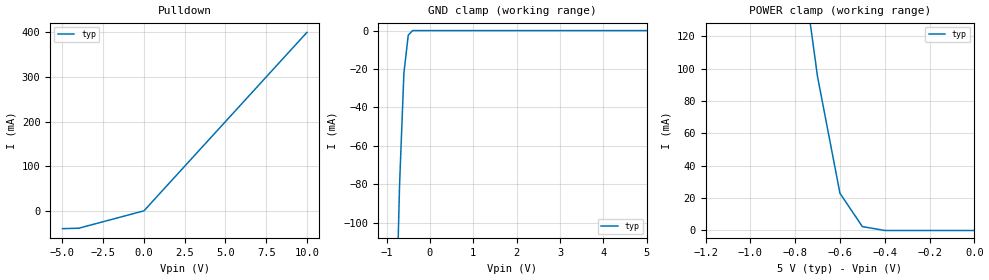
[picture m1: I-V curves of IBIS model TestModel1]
[IBIS Ver]   3.2
[File Name]   bug54b.ibs
[File Rev]   0.0
[Date]   22-February-2001
[Source]   File created from specification
[Notes]   Using the IBISCHK3 v3.2.5 & v3.2.6 parsers, the
   following file will show two misleading warnings
   related to the buffer delay fixture.
[Disclaimer]
   (C) Copyright 2001 Intel Corp.
   All rights reserved
   This model is for demonstration purposes only,
[Component]   GENERIC_IBIS
[Manufacturer]   Intel Corp.
[Package]
|   typ   min   max
R_pkg   6.0mO   5.0mO   7.0mO
L_pkg   5.0nH   2.0nH   8.0nH
C_pkg   1.0pF   0.5pF   1.5pF
[Pin]   signal_name   model_name   R_pin   L_pin   C_pin
   1   TestSignal1   TestModel1
| Models and submodels in the file (1): TestModel1 (I/O_open_sink)
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[Model]   TestModel1
Model_type   I/O_open_sink
| Model_type   I/O
Polarity   Non-Inverting
Enable   Active-Low
Vinl = 800mV
Vinh = 2.0V
Cref  = 0F
Rref  = 25ohms
Vref  = 5.0V
Vmeas = 2.5V
C_comp   5.00pF   4.00pF   6.00pF
[Temperature Range]   27.00   100.00   0.00
[Voltage Range]   5.0V   4.75V   5.25V
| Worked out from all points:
|   slope of the pulldown table from 0 to 0.75 V, typ, clamps not added: 25 ohm
|   GND clamp passes 1 mA (typ) near -0.44 V on its own axis
|   POWER clamp passes 1 mA (typ) near -0.44 V on its own axis
[Pullup]
| voltage   I(typ)   I(min)   I(max)
-5V       0A         NA         NA
-4V       0A         NA         NA
0V        0A         NA         NA
5V        0A         NA         NA
10V       0A         NA         NA
[Pulldown]
| voltage   I(typ)   I(min)   I(max)
-5V       -40mA      NA         NA
-4V       -39mA      NA         NA
0V        0A         NA         NA
5V        200mA      NA         NA
10V       400mA      NA         NA
[GND Clamp]
| voltage   I(typ)   I(min)   I(max)
-5V       -3.9A      NA         NA
-700mV    -80mA      NA         NA
-600mV    -22mA      NA         NA
-500mV    -2.4mA     NA         NA
-400mV    0A         NA         NA
5V        0A         NA         NA
[Power Clamp]
| voltage   I(typ)   I(min)   I(max)
-5V       4.45A      NA         NA
-700mV    95mA       NA         NA
-600mV    23mA       NA         NA
-500mV    2.4mA      NA         NA
-400mV    0A         NA         NA
0V        0A         NA         NA
[Ramp]
|variable   typ   min   max
dV/dt_r   2.20/1.06n   1.92/1.28n   2.49/650p
dV/dt_f   2.46/1.21n   2.21/1.54n   2.70/770p
R_load = 300ohms
